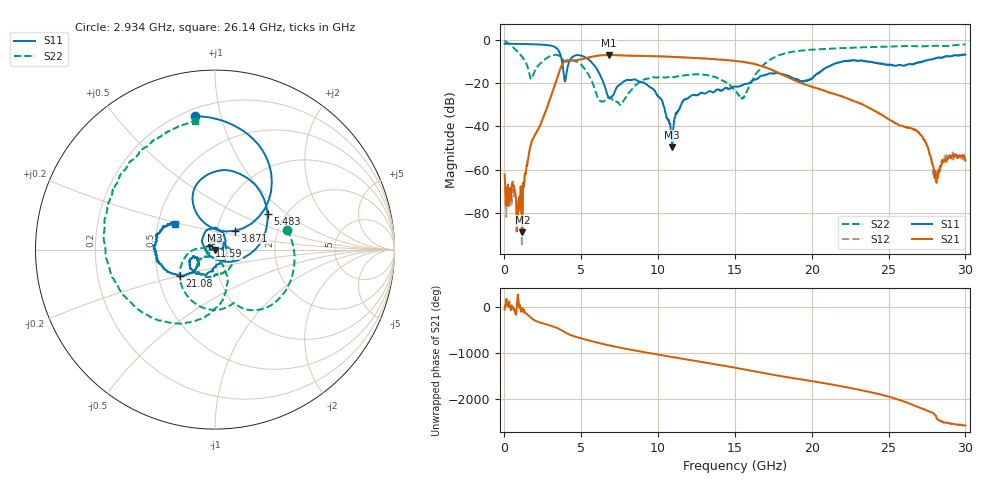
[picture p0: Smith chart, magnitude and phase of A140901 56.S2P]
!  2-Port S-parameters saved by WinCal
! VAR MeasName=S-Parameters (CALIBRATED_DATA) read from VNA (N5244A)
! VAR MeasDate=11/3/2014 9:36:16 AM
! VAR NAME=A140901 56
! VAR FILENAME=A140901 56.S2P
! VAR DATE=11/3/2014 9:36:17 AM
! VAR PHYS_PORTS=1,2
# Hz S RI R 50
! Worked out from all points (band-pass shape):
!   801 points, 10 MHz to 30 GHz, reference 50 ohm
!   highest |S21| = -6.94 dB at 6.795 GHz (marker M1); lowest = -89.0 dB at 1.172 GHz (marker M2)
!   |S21| within 3 dB of the highest: 3.899 GHz to 15.33 GHz (11.43 GHz wide, 119 % of centre)
!   lowest |S11| = -49.6 dB at 10.92 GHz (marker M3), VSWR 1.01, Z = 49.8 - j0.217 ohm
!   |S11| at or under -10 dB: 3.749 GHz to 4.217 GHz (468.2 MHz wide, 11.8 % of centre); 5.631 GHz to 21.97 GHz (16.33 GHz wide, 118 % of centre); 23.83 GHz to 27.23 GHz (3.407 GHz wide, 13.3 % of centre)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
!   |S22| runs from -30.1 to -0.2 dB; largest |S21 - S12| = 0.0031
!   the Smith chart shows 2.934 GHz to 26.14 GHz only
!   S11 on the Smith chart (normalised r, x): 2.934 GHz: 0.24, +0.83; 3.871 GHz: 1.22, +0.26; 5.483 GHz: 1.63, +0.73; 11.59 GHz: 0.94, +0.04; 21.08 GHz: 0.65, -0.20; 26.14 GHz: 0.61, +0.19
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1e7  -0.8184 0.00136  0.000453 -0.00063  -0.000115 -0.000262  0.9771 -0.0346
5.34825e8  -0.7984 0.1736  0.000415 4.2e-05  0.000485 -0.000231  0.238 -0.6544
1.172112e9  -0.7205 0.3695  3.28e-05 -1.36e-05  5.41e-05 -4.94e-05  -0.3403 -0.2068
1.734425e9  -0.6013 0.5268  -0.00214 0.0033  -0.00228 0.00334  -0.1031 0.0695
2.934025e9  -0.1095 0.7433  0.0318 -0.0241  0.0316 -0.0241  0.4003 0.1101
3.871212e9  0.1112 0.1053  -0.3105 -0.0248  -0.3098 -0.0249  0.1204 -0.3075
5.033325e9  0.2041 0.3795  0.288 0.216  0.2874 0.2163  -0.1943 -0.169
5.483175e9  0.2935 0.1973  0.3944 -0.0196  0.3942 -0.0188  -0.1528 -0.0249
6.795238e9  -0.0171 -0.0424  -0.1519 -0.4234  -0.1513 -0.4231  -0.0436 -0.0157
8.069812e9  -0.0354 0.1149  -0.4198 0.1152  -0.4196 0.1147  0.0495 0.0298
1.001916e10  0.0456 0.0167  0.2756 0.3176  0.2749 0.3169  0.0442 -0.129
1.091886e10  -0.00248 -0.00219  0.4076 -0.0136  0.4068 -0.0135  0.00964 -0.1372
1.159364e10  -0.031 0.0192  0.3061 -0.2525  0.306 -0.2526  -0.0145 -0.1487
1.5005e10  0.0229 -0.0799  -0.1997 0.2611  -0.2007 0.261  -0.0546 -0.0403
1.676691e10  -0.0523 -0.1418  0.2361 0.0776  0.2357 0.0775  0.0602 -0.236
2.002832e10  -0.0961 -0.0882  -0.0793 -0.0227  -0.0793 -0.0239  -0.5862 -0.1101
2.107798e10  -0.1951 -0.1464  -0.0443 0.0427  -0.0453 0.0431  -0.617 0.1015
2.501416e10  -0.2182 0.1493  -0.0109 -0.00968  -0.011 -0.00975  -0.2728 0.6526
2.613879e10  -0.2252 0.1435  -0.00138 0.00958  -0.00159 0.00959  -0.11 0.7174
2.73009e10  -0.2707 0.1769  0.00328 -0.00361  0.00322 -0.00408  0.0442 0.7163
2.812562e10  -0.2849 0.2557  -0.000152 0.000471  -0.000499 0.000762  0.1485 0.7207
3e10  -0.1988 0.4156  0.00125 -0.00102  0.00103 -0.0012  0.3682 0.7039
